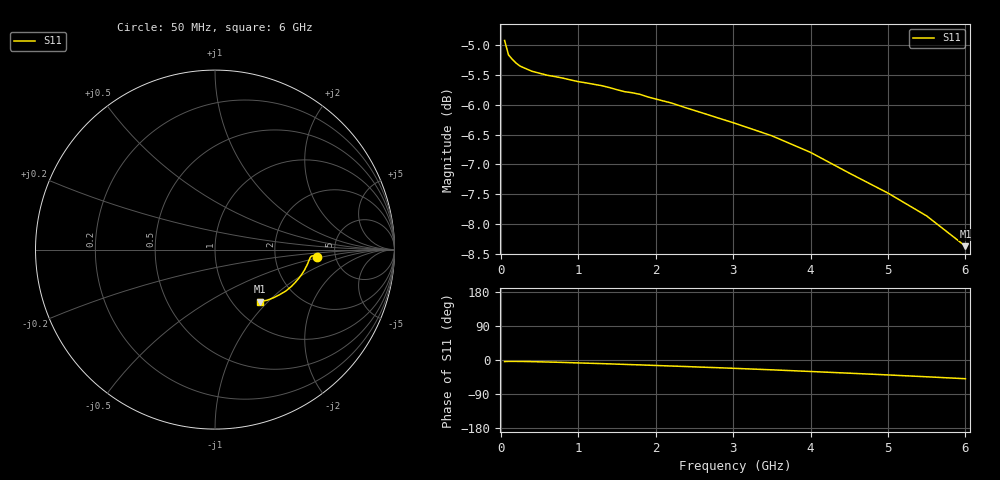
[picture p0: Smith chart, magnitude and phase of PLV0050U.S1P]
! Infineon Technologies  Discrete & RF Semiconductors
! BAR 64-04W /-05W /-06W
! Si PIN Diode in SOT323
! IF = 0.05 mA
! S-Parameters:  October  2008
# GHz  S  MA  R  50
!  f  S11
! GHz  MAG  ANG
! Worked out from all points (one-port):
!   34 points, 50 MHz to 6 GHz, reference 50 ohm
!   lowest |S11| = -8.4 dB at 6 GHz (marker M1), VSWR 2.23, Z = 65.8 - j44.6 ohm
!   |S11| at or under -10 dB: nowhere
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0.05  0.5676 -4.1
0.1  0.552 -3.6
0.15  0.5473 -3.6
0.2  0.5432 -3.7
0.25  0.5401 -3.8
0.3  0.5384 -3.9
0.4  0.5349 -4.3
0.6  0.5307 -5.3
0.7  0.5293 -5.8
0.8  0.5278 -6.4
0.9  0.526 -7.0
1  0.5242 -7.7
1.3  0.5202 -9.5
1.6  0.5141 -11.6
1.7  0.5131 -12.3
1.8  0.5114 -12.9
1.9  0.5089 -13.7
2.2  0.5031 -15.9
2.4  0.4981 -17.3
2.6  0.4935 -18.9
2.8  0.4888 -20.3
3  0.4842 -21.9
3.5  0.4721 -25.9
4  0.4572 -30.3
4.5  0.4393 -34.8
5  0.4226 -39.4
5.5  0.4043 -44.3
6  0.3814 -49.4
